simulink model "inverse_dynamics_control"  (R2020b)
settings: Solver=VariableStepAuto  StartTime=0.0  StopTime=10.0  RelTol=1e-3
undefined symbols (not defined in the file or in its folder): B, Spline
libraries: robotcorelib x1, simulink x1

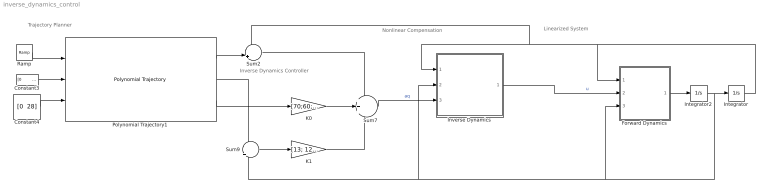
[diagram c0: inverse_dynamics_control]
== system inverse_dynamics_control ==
  note: Trajectory Planner
  note: Nonlinear Compensation
  note: Linearized System
  note: Inverse Dynamics Controller
  Constant3 : Constant  Value="[0         0    2.1340    3.1416    4.3901    5.3086    6.2832; 0.1992   -0.6287   -1.4202   -1.5337   -1.4017   -1.4251   -0.8779; -1.3608    1.1882    2.9776    2.6877    2.8054    2.9089    1.5527; 0         0    1.5535         0    1.5621    1.6822    3.1416;0.4092    2.1303    1.1005   -0.3049   -1.3946   -2.3249   -2.2457;0         0   -1.5677   -3.1416   -1.7353   -1.7086   -3.1416]"
  Constant4 : Constant  Value="[0  28]"  VectorParams1D=off
  Forward Dynamics : MATLAB Function  TreatAsAtomicUnit=on
  Integrator : Integrator  InitialCondition=[0;0;0;0;0;0]  AbsoluteTolerance=1e-10
  Integrator2 : Integrator  InitialCondition=[0;0;0;0;0;0]  AbsoluteTolerance=1e-10
  Inverse Dynamics : MATLAB Function  TreatAsAtomicUnit=on
  K0 : Gain  Gain=[70;60;20;5;5;5]
  K1 : Gain  Gain=[13; 12; 5; 3.8; 3; 3]
  Polynomial Trajectory1 : robotcorelib/Polynomial Trajectory  WaypointSource=External  Waypoints=[ 0, 2, 1, 5, 0; -1, 3, 1, 4, 4 ]  TimePoints=[ 0, 1, 2, 3, 4 ]  TimeInterval=[ 1, 4 ]  Method=B-Spline  ParameterSource=Internal  VelocityBoundaryCondition=zeros( 2, 5 )  AccelerationBoundaryCondition=zeros( 2, 5 )  SimulateUsing=Interpreted execution
  Ramp : simulink/Sources/Ramp  slope=1  start=0  InitialOutput=0
  Sum2 : Sum  Inputs=-|+||
  Sum7 : Sum  Inputs=+++
  Sum9 : Sum  Inputs=-||+
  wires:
  K1/1 -> Sum7/3
  Polynomial Trajectory1/2 -> Sum9/1
  Ramp/1 -> Polynomial Trajectory1/1
  Polynomial Trajectory1/3 -> K0/1
  Constant4/1 -> Polynomial Trajectory1/3
  Constant3/1 -> Polynomial Trajectory1/2
  Polynomial Trajectory1/1 -> Sum2/2
  Integrator2/1 -> Integrator/1, Forward Dynamics/3(dq), Sum9/2, Inverse Dynamics/2(dq)
  Sum9/1 -> K1/1
  K0/1 -> Sum7/2
  Sum2/1 -> Sum7/1
  Sum7/1 -> Inverse Dynamics/3(aq)  "aq"
  Inverse Dynamics/1(u) -> Forward Dynamics/2(u)  "u"
  Forward Dynamics/1(ddq) -> Integrator2/1
  Integrator/1 -> Inverse Dynamics/1(q), Sum2/1, Forward Dynamics/1(q)

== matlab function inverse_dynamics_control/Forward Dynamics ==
function ddq = fcn(q,u,dq)

ddq = zeros(6,1); %added to help simulink


gz = 9.81;
U_F = 1;
m = [1.25 1.55 1.98 1.14 1.14 1.03 1];

[M,Cdq,G,N_D,G_B] = getDCGfunc_v4([q,dq],m,gz,U_F);
    
ddq = M\(-Cdq - G - N_D - G_B + u );

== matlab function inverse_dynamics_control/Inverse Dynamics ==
function u = fcn(q,dq,aq)

u = zeros(6,1); %added to help simulink

gz = 9.81;
U_F = 1;
m = [1.35 1.65 2.08 1.24 1.24 1.13 1];


[M,Cdq,G,N_D,G_B] = getDCGfunc_v4([q,dq],m,gz,U_F);
    
u = M*aq + Cdq + G + N_D + G_B;
